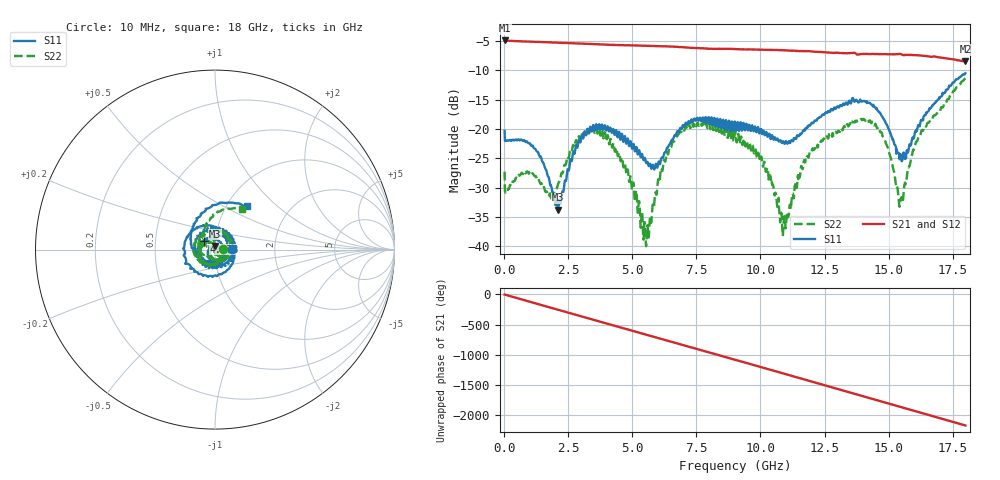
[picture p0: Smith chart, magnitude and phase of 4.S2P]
!Agilent Technologies,E5071C,MY46316741,A.11.02
!Date: Tue Sep 22 10:34:13 2020
!Data & Calibration Information:
!Freq	S11:SOLT4(ON)	S21:SOLT4(ON)	S12:SOLT4(ON)	S22:SOLT4(ON)
!PortZ  Port1:50+j0  Port2:50+j0
!Above PortZ is port z conversion or system Z0 setting when saving the data.
!When reading, reference impedance value at option line is always used.
# Hz S dB R 50
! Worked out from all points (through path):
!   1561 points, 10 MHz to 18 GHz, reference 50 ohm
!   highest |S21| = -4.92 dB at 10 MHz (marker M1); lowest = -8.5 dB at 18 GHz (marker M2)
!   group delay of S21, straight-line fit = 335 ps
!   lowest |S11| = -33.7 dB at 2.097 GHz (marker M3), VSWR 1.04, Z = 49.7 + j2.03 ohm
!   |S11| at or under -10 dB: start of sweep to end of sweep
!   |S22| runs from -40.0 to -11.4 dB; largest |S21 - S12| = 0.014
!   S11 on the Smith chart (normalised r, x): 10 MHz: 1.21, +0.01; 4.773 GHz: 0.88, +0.08; 18 GHz: 1.24, +0.65
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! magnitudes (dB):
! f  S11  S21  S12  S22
! 10 MHz  -20.3  -4.9  -4.9  -27.3
! 1.255 GHz  -23.8  -5.2  -5.2  -28.3
! 1.786 GHz  -29.4  -5.2  -5.2  -31.0
! 2.097 GHz  -33.7  -5.3  -5.3  -29.4
! 3.02 GHz  -21.0  -5.4  -5.5  -20.6
! 3.862 GHz  -20.1  -5.6  -5.6  -21.6
! 4.773 GHz  -22.4  -5.7  -5.8  -27.7
! 5.488 GHz  -25.0  -5.8  -5.8  -36.0
! 6.007 GHz  -25.8  -5.9  -5.9  -28.6
! 6.514 GHz  -22.1  -6.0  -6.0  -23.1
! 7.137 GHz  -19.3  -6.1  -6.1  -20.0
! 9.005 GHz  -18.8  -6.4  -6.4  -20.5
! 10.1 GHz  -20.4  -6.5  -6.5  -26.4
! 10.92 GHz  -22.4  -6.6  -6.6  -34.9
! 11.53 GHz  -21.0  -6.7  -6.7  -28.2
! 12.01 GHz  -18.9  -6.8  -6.8  -23.5
! 13.98 GHz  -15.3  -7.2  -7.2  -18.5
! 14.55 GHz  -16.7  -7.2  -7.3  -19.9
! 15 GHz  -20.0  -7.3  -7.3  -23.8
! 15.49 GHz  -24.9  -7.2  -7.3  -31.8
! 16.24 GHz  -19.1  -7.5  -7.5  -21.1
! 18 GHz  -10.5  -8.5  -8.5  -11.4
